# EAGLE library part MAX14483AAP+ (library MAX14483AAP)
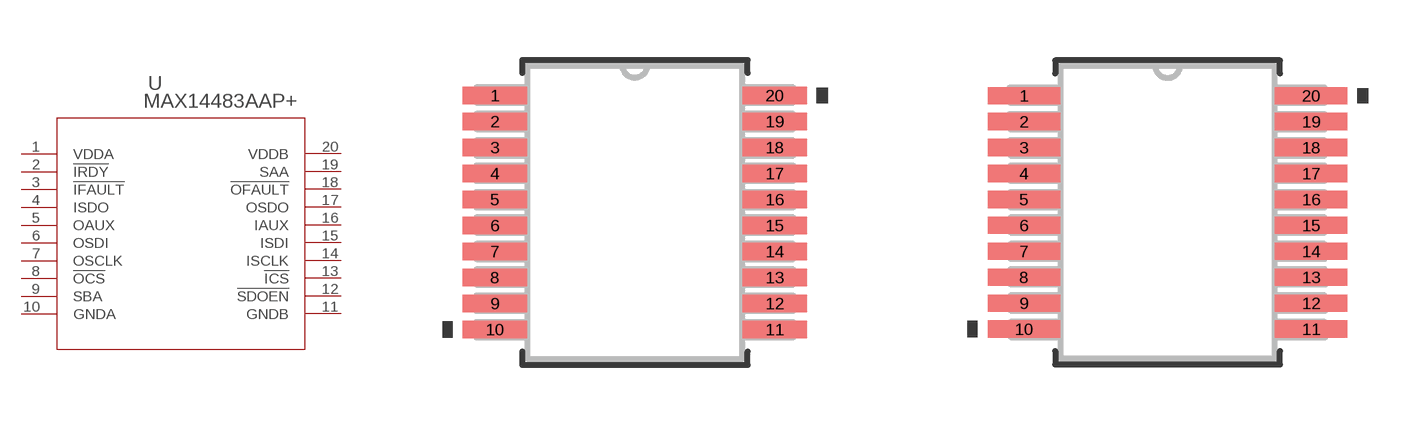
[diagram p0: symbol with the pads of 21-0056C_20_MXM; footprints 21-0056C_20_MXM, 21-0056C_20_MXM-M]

Designator prefix U

## MAX14483AAP+ (COPYRIGHT: Copyright (C) 2022 Ultra Librarian. All rights reserved.; MANUFACTURER_PART_NUMBER: MAX14483AAP+; MFR_NAME: Maxim Integrated Products)  [21-0056C_20_MXM]
1  VDDA  pwr
2  !IRDY  pas
3  !IFAULT  pas
4  ISDO  pas
5  OAUX  pas
6  OSDI  pas
7  OSCLK  pas
8  !OCS  pas
9  SBA  pas
10  GNDA  pas
11  GNDB  pas
12  !SDOEN  pas
13  !ICS  pas
14  ISCLK  pas
15  ISDI  pas
16  IAUX  pas
17  OSDO  pas
18  !OFAULT  pas
19  SAA  pas
20  VDDB  pwr

## MAX14483AAP+21-0056C_20_MXM-M (COPYRIGHT: Copyright (C) 2022 Ultra Librarian. All rights reserved.; MANUFACTURER_PART_NUMBER: MAX14483AAP+; MFR_NAME: Maxim Integrated Products)  [21-0056C_20_MXM-M]
Pads as for 21-0056C_20_MXM

## MAX14483AAP+21-0056C_20_MXM-L (COPYRIGHT: Copyright (C) 2022 Ultra Librarian. All rights reserved.; MANUFACTURER_PART_NUMBER: MAX14483AAP+; MFR_NAME: Maxim Integrated Products)  [21-0056C_20_MXM-L]
Pads as for 21-0056C_20_MXM

## Footprint 21-0056C_20_MXM (pad centres in mm)
smd 1.613 x 0.432: 1 -3.499,2.925; 2 -3.499,2.275; 3 -3.499,1.625; 4 -3.499,0.975; 5 -3.499,0.325; 6 -3.499,-0.325; 7 -3.499,-0.975; 8 -3.499,-1.625; 9 -3.499,-2.275; 10 -3.499,-2.925; 11 3.499,-2.925; 12 3.499,-2.275; 13 3.499,-1.625; 14 3.499,-0.975; 15 3.499,-0.325; 16 3.499,0.325; 17 3.499,0.975; 18 3.499,1.625; 19 3.499,2.275; 20 3.499,2.925

## Footprint 21-0056C_20_MXM-M (pad centres in mm)
smd 1.816 x 0.432: 1 -3.6,2.925; 2 -3.6,2.275; 3 -3.6,1.625; 4 -3.6,0.975; 5 -3.6,0.325; 6 -3.6,-0.325; 7 -3.6,-0.975; 8 -3.6,-1.625; 9 -3.6,-2.275; 10 -3.6,-2.925; 11 3.6,-2.925; 12 3.6,-2.275; 13 3.6,-1.625; 14 3.6,-0.975; 15 3.6,-0.325; 16 3.6,0.325; 17 3.6,0.975; 18 3.6,1.625; 19 3.6,2.275; 20 3.6,2.925

## Footprint 21-0056C_20_MXM-L (pad centres in mm)
smd 1.346 x 0.381: 1 -3.429,2.925; 2 -3.429,2.275; 3 -3.429,1.625; 4 -3.429,0.975; 5 -3.429,0.325; 6 -3.429,-0.325; 7 -3.429,-0.975; 8 -3.429,-1.625; 9 -3.429,-2.275; 10 -3.429,-2.925; 11 3.429,-2.925; 12 3.429,-2.275; 13 3.429,-1.625; 14 3.429,-0.975; 15 3.429,-0.325; 16 3.429,0.325; 17 3.429,0.975; 18 3.429,1.625; 19 3.429,2.275; 20 3.429,2.925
